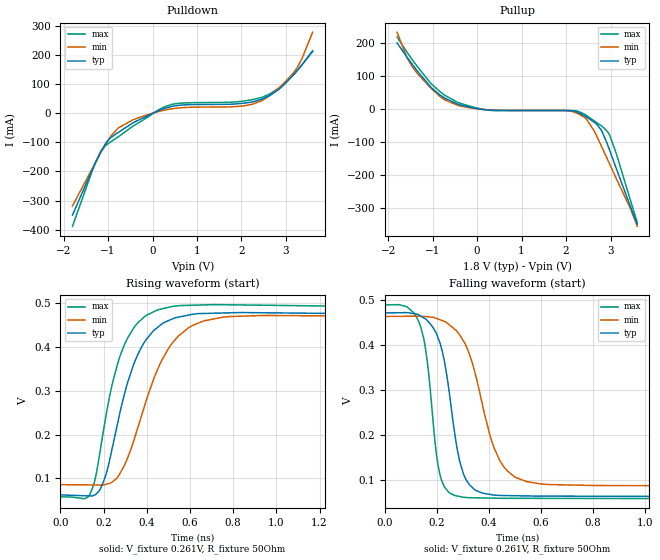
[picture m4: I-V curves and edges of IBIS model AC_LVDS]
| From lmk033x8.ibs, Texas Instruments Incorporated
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[Model]   AC_LVDS
Model_type   Output
Polarity   Non-Inverting
Vmeas = 0.9
Vref = 1.8
Cref = 15pF
Rref = 50
|   typ   min   max
|   (nom PVT)   (fast PVT)   (slow PVT)
C_comp   0.989p   0.973p   0.998p
|C_comp (ON state)   0.989p   0.973p   0.998p
|C_comp (OFF state)   0.989p   0.973p   0.998p
| Where   nom PVT is  Nominal Process, 1.8V, 27C
|   Fast PVT is Strong Process, 1.9V, -40C
|   Slow PVT is Weak Process, 1.7V, 125C
[Voltage Range]   1.8   1.7   1.9
[Temperature Range]   27   125   -40
[Pullup Reference]   1.8   1.7   1.9
[Pulldown Reference]   0   0   0
[Power Clamp Reference]   1.8   1.7   1.9
[GND Clamp Reference]   0   0   0
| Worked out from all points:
|   slope of the pulldown table from 0 to 0.27 V, typ, clamps not added: 15.8 ohm
|   slope of the pullup table from 0 to 0.27 V, typ, clamps not added: 58 ohm
|   falling waveform, V_fixture 0.261V, R_fixture 50Ohm: 20-80 % time 67.8ps typ, 108ps min, 48.5ps max; typ from 0.471 V to 0.062 V
|   rising waveform, V_fixture 0.261V, R_fixture 50Ohm: 20-80 % time 136ps typ, 168ps min, 117ps max; typ from 0.062 V to 0.471 V
[Pulldown]
|   Voltage   I(typ)   I(min)   I(max)
-1.8V     -350mA     -318.8mA   -388.5mA
-1.282V   -169.2mA   -169mA     -170.1mA
-1.028V   -98.31mA   -99.9mA    -107.8mA
-763.2mV  -65.13mA   -50.09mA   -80.46mA
-444.6mV  -33.56mA   -23.1mA    -45.01mA
387mV     21.51mA    13.95mA    28.19mA
1.975V    33.17mA    24.09mA    40.37mA
2.455V    48.03mA    42.94mA    54.23mA
2.849V    82.71mA    88.09mA    86.71mA
3.168V    131.8mA    138.3mA    131mA
3.357V    165.6mA    185.9mA    165.1mA
3.6V      212.1mA    278mA      214.6mA
[Pullup]
|   Voltage   I(typ)   I(min)   I(max)
-1.8V     201.2mA    233.7mA    219.3mA
-1.579V   158.5mA    156.6mA    173.5mA
-1.444V   133.5mA    125.8mA    147.6mA
-1.049V   68.37mA    65.07mA    79.96mA
-730.8mV  33.76mA    28.59mA    42.46mA
241.2mV   -2.873mA   -2.188mA   -2.848mA
2.104V    -4.67mA    -6.288mA   -4.57mA
2.461V    -24.42mA   -30.6mA    -19.3mA
2.671V    -43.29mA   -77.22mA   -39.59mA
2.806V    -67.6mA    -115.8mA   -52.1mA
2.984V    -126.6mA   -168.4mA   -80.59mA
3.6V      -349.9mA   -356.5mA   -344.6mA
[Ramp]
R_load = 50
|   typ   min   max
dV/dt_r   0.245383/1.35469e-10   0.226741/1.67045e-10   0.258883/1.16535e-10
dV/dt_f   0.245383/6.7437e-11   0.226741/1.07142e-10   0.258883/4.8188e-11
[Falling Waveform]
V_fixture = 0.261V
V_fixture_min = 0.272V
V_fixture_max = 0.263V
R_fixture = 50Ohm
C_fixture = 0F
|   Time   V(typ)   V(min)   V(max)
0s        471.2mV    463.4mV    489.2mV
134.6ps   465.1mV    464mV      444.5mV
162.8ps   454.1mV    462.7mV    361.8mV
195.2ps   427.9mV    459.5mV    168.8mV
228.2ps   364.2mV    452.4mV    84.03mV
274.4ps   178.3mV    431.6mV    64.04mV
302.1ps   112.4mV    408.2mV    60.75mV
441.6ps   64.78mV    142.6mV    58.54mV
611.8ps   63.29mV    89.86mV    58.3mV
6.7ns     62.18mV    85.5mV     57.69mV
[Rising Waveform]
V_fixture = 0.261V
V_fixture_min = 0.272V
V_fixture_max = 0.263V
R_fixture = 50Ohm
C_fixture = 0F
|   Time   V(typ)   V(min)   V(max)
0s        62.18mV    85.5mV     57.69mV
138ps     59.66mV    84.97mV    65.14mV
164.9ps   63.93mV    84.86mV    108.1mV
202.3ps   96.23mV    85.23mV    218mV
263.5ps   222.5mV    101.7mV    359mV
375.5ps   399.7mV    243mV      463mV
519.5ps   464.2mV    409.9mV    492.7mV
665.8ps   476.5mV    459.8mV    496mV
943.2ps   478mV      471.9mV    495.3mV
6.7ns     471.2mV    463.4mV    489.2mV
